(* Logix 5000 AddOnInstructionDefinition export; software revision 16.04 *)

TYPE AKD_Status :   // All connections to the drive ethernet module are established and data is successfully transferring.
STRUCT
   Profile_In_Progress : BOOL;   // Profile Move In Progress
   Block_In_Execution : BOOL;   // Block In Execution
   On_Target_Position : BOOL;   // On Target Position (1=Current Position Equals Last Target Position)
   General_Fault : BOOL;   // General Fault
   Current_Direction : BOOL;   // Current Motor Direction (0=Reverse, 1=Forward)
   Home_Level : BOOL;   // Level of Home Input
   Reg_Level : BOOL;   // Level of Registration Input
   Enable : BOOL;   // State of Enable Output
   Fault_Input_Fault : BOOL;   // Fault Input Active
   Fwd_Limit : BOOL;   // Forward Input Active
   Rev_Limit : BOOL;   // Reverse Input Active
   Positive_Limit : BOOL;   // Positive Software Limit Exceeded
   Negative_Limit : BOOL;   // Negative Software Limit Exceeded
   FE_Fault : BOOL;   // Following Error Fault
   Block_Fault : BOOL;   // Block Execution Fault
   Load_Complete : BOOL;   // Command Message Successfully Loaded
END_STRUCT
END_TYPE

TYPE AKD_Axis :   // Axis Data:
STRUCT
   Control : AKD_Control;   // Control bits to send to the drive
   Status : AKD_Status;   // Status bits received from the drive
   Input : AB:ETHERNET_MODULE_SINT_64Bytes:I:0;   // Data from the drive
   Output : AB:ETHERNET_MODULE_SINT_64Bytes:O:0;   // Data to the drive
   ResponseMsgType : SINT;   // Response type contained in latest IO response from drive. Used to check for errors
   CommandTimeout : INT;   // Time to allow for command response from drive. Dependent on scan rate and communicaiton rate
   PositionFeedback : DINT;   // Actual Position Value
   VelocityFeedback : DINT;   // Actual Velocity Value
END_STRUCT
END_TYPE

TYPE AKD_Control :   // Send Explicit Message
STRUCT
   Load_Data_Start_Profile : BOOL;   // Load Command Data / Start Profile Move
   Start_Block : BOOL;   // Execute Command block or block chain
   Incremental : BOOL;   // Incremental Position (0=Absolute, 1=Incremental)
   Direction : BOOL;   // Direction in Velocity Mode (0=Reverse, 1=Forward)
   Smooth_Stop : BOOL;   // Smooth / Controlled Stop w/ Deceleration
   Hard_Stop : BOOL;   // Hard / Immediate Stop
   Reg_Arm : BOOL;   // Arm the Registration Input
   Enable : BOOL;   // Enable Output
END_STRUCT
END_TYPE

ADD_ON_INSTRUCTION AKD_Set_Position   (* revision 2.1, ExecutePrescan, ExecuteEnableInFalse *)
// Set Drive Position
// Revision note:
// Don't error if Command_Timeout preset is 0
VAR_OUTPUT
   DN : BOOL; {visible}   // Command Successful
   ER : BOOL; {visible}   // Error
END_VAR
VAR_IN_OUT
   Axis : AKD_Axis; {required}
END_VAR
VAR_INPUT
   Incremental : BOOL; {visible}   // Position Definition (0=Absolute, 1=Incremental)
   Position : DINT; {required}   // Position Value
END_VAR
VAR_OUTPUT
   PC : BOOL; {visible}   // Process Complete
   IP : BOOL; {visible}   // In Process
END_VAR
VAR
   Response_Bytes : SINT[8];
   OS_LoadStart : BOOL;
   Position_Internal : DINT;   // Scaled Position Value for Drive
   Command_Timeout : TIMER;   // Timeout Timer
   Command_Message_Type : SINT;   // Command Message Type
   Command_Axis_Number : SINT;   // Command Axis Number
   Response_Message_Type : SINT;   // Response Message Type
   Response_Axis_Number : SINT;   // Response Axis Number
   Command_Bytes : SINT[8];
   Step : SINT;
END_VAR

ROUTINE EnableInFalse   (* ladder *)
// EnableIn_False
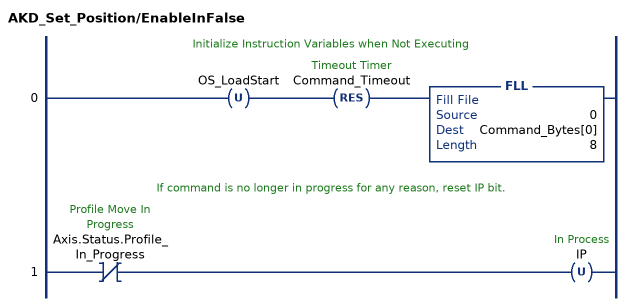
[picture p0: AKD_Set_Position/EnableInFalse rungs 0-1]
   // Initialize Instruction Variables when Not Executing
   0: OTU(OS_LoadStart)RES(Command_Timeout)FLL(0,Command_Bytes[0],8);
   // If command is no longer in progress for any reason, reset IP bit.
   1: XIO(Axis.Status.Profile_In_Progress)OTU(IP);
END_ROUTINE

ROUTINE Logic   (* ladder *)
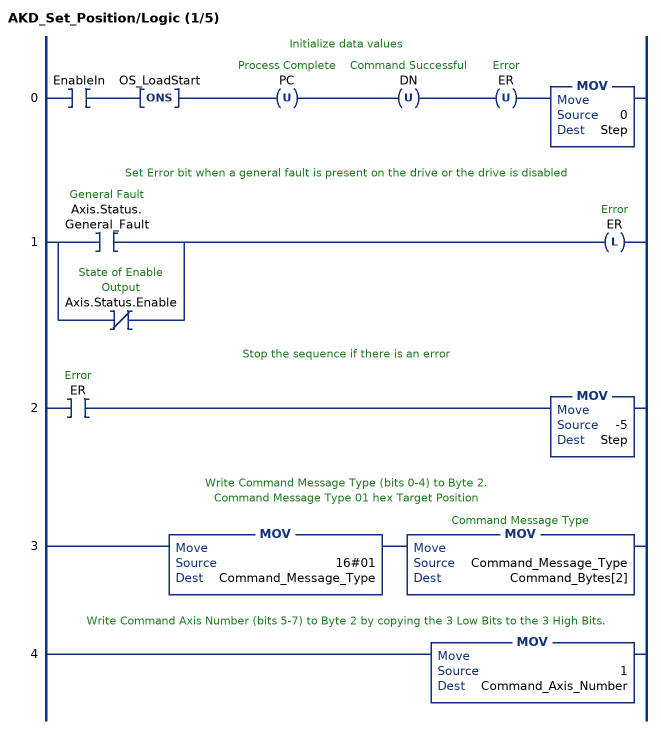
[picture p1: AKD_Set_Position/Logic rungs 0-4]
   // Initialize data values
   0: XIC(EnableIn)ONS(OS_LoadStart)OTU(PC)OTU(DN)OTU(ER)MOV(0,Step);
   // Set Error bit when a general fault is present on the drive or the drive is disabled
   1: [XIC(Axis.Status.General_Fault) ,XIO(Axis.Status.Enable) ]OTL(ER);
   // Stop the sequence if there is an error
   2: XIC(ER)MOV(-5,Step);
   // Write Command Message Type (bits 0-4) to Byte 2.
   // Command Message Type 01 hex Target Position
   3: MOV(16#01,Command_Message_Type)MOV(Command_Message_Type,Command_Bytes[2]);
   // Write Command Axis Number (bits 5-7) to Byte 2 by copying the 3 Low Bits to the 3 High Bits.
   4: MOV(1,Command_Axis_Number);
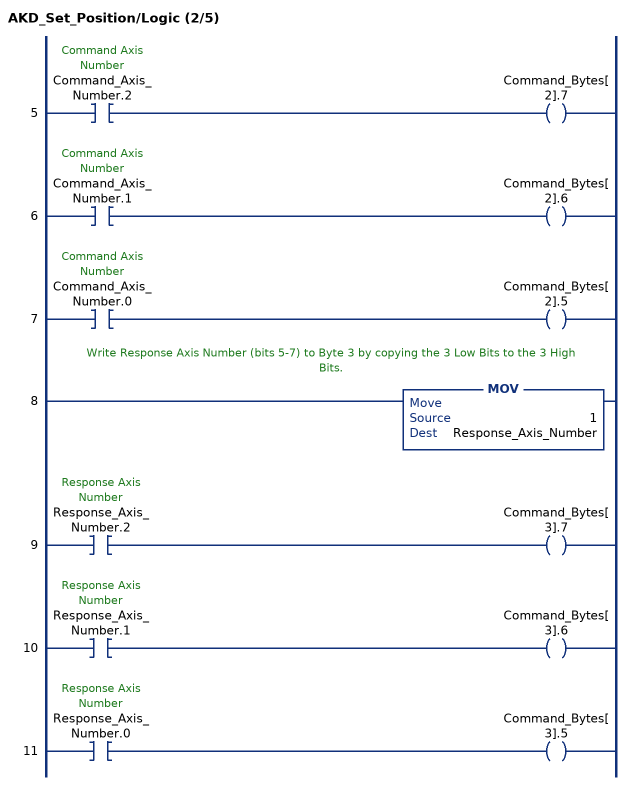
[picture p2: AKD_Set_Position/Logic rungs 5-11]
   5: XIC(Command_Axis_Number.2)OTE(Command_Bytes[2].7);
   6: XIC(Command_Axis_Number.1)OTE(Command_Bytes[2].6);
   7: XIC(Command_Axis_Number.0)OTE(Command_Bytes[2].5);
   // Write Response Axis Number (bits 5-7) to Byte 3 by copying the 3 Low Bits to the 3 High Bits.
   8: MOV(1,Response_Axis_Number);
   9: XIC(Response_Axis_Number.2)OTE(Command_Bytes[3].7);
   10: XIC(Response_Axis_Number.1)OTE(Command_Bytes[3].6);
   11: XIC(Response_Axis_Number.0)OTE(Command_Bytes[3].5);
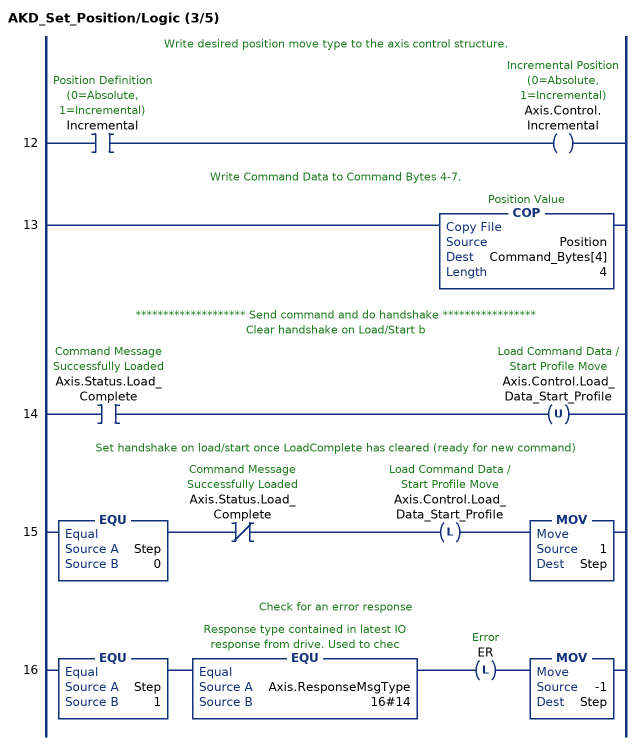
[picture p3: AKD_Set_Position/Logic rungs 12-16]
   // Write desired position move type to the axis control structure.
   12: XIC(Incremental)OTE(Axis.Control.Incremental);
   // Write Command Data to Command Bytes 4-7.
   13: COP(Position,Command_Bytes[4],4);
   // ******************** Send command and do handshake *****************
   // Clear handshake on Load/Start b
   14: XIC(Axis.Status.Load_Complete)OTU(Axis.Control.Load_Data_Start_Profile);
   // Set handshake on load/start once LoadComplete has cleared (ready for new command)
   15: EQU(Step,0)XIO(Axis.Status.Load_Complete)OTL(Axis.Control.Load_Data_Start_Profile)MOV(1,Step);
   // Check for an error response
   16: EQU(Step,1)EQU(Axis.ResponseMsgType,16#14)OTL(ER)MOV(-1,Step);
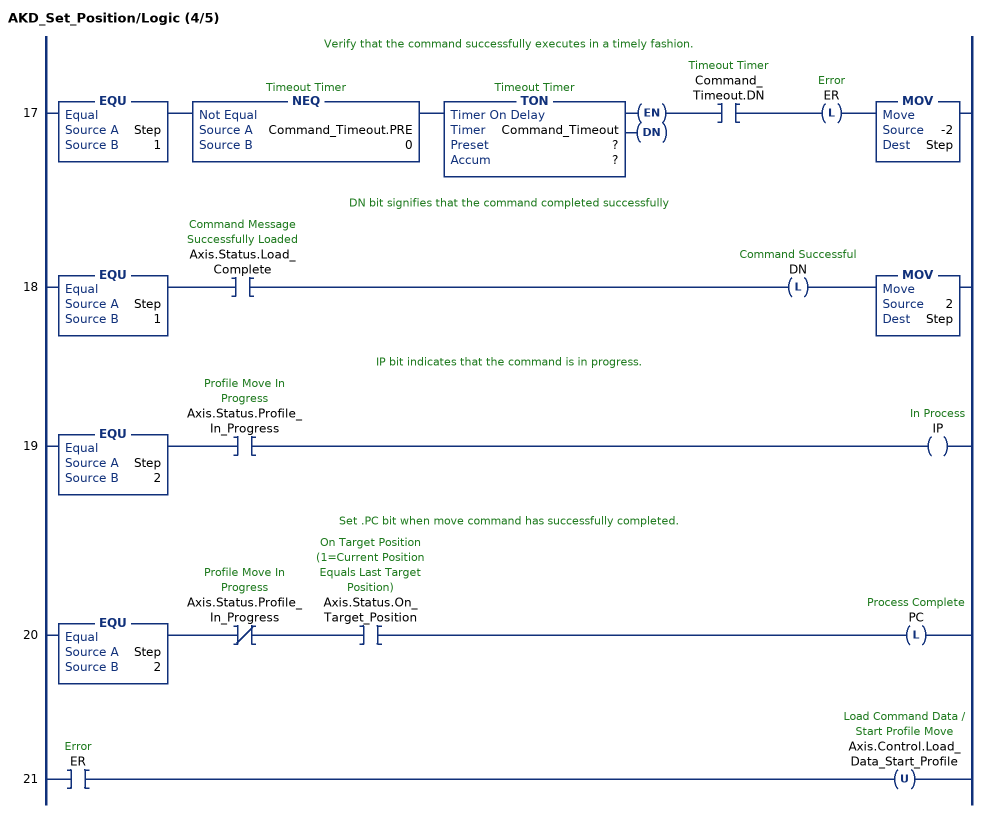
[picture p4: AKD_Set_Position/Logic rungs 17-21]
   // Verify that the command successfully executes in a timely fashion.
   17: EQU(Step,1)NEQ(Command_Timeout.PRE,0)TON(Command_Timeout,?,?)XIC(Command_Timeout.DN)OTL(ER)MOV(-2,Step);
   // DN bit signifies that the command completed successfully
   18: EQU(Step,1)XIC(Axis.Status.Load_Complete)OTL(DN)MOV(2,Step);
   // IP bit indicates that the command is in progress.
   19: EQU(Step,2)XIC(Axis.Status.Profile_In_Progress)OTE(IP);
   // Set .PC bit when move command has successfully completed.
   20: EQU(Step,2)XIO(Axis.Status.Profile_In_Progress)XIC(Axis.Status.On_Target_Position)OTL(PC);
   21: XIC(ER)OTU(Axis.Control.Load_Data_Start_Profile);
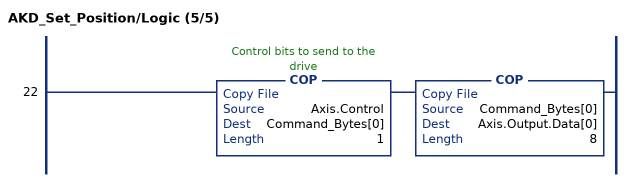
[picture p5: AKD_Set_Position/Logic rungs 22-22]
   22: COP(Axis.Control,Command_Bytes[0],1)COP(Command_Bytes[0],Axis.Output.Data[0],8);
END_ROUTINE

ROUTINE Prescan   (* ladder *)
// Prescan
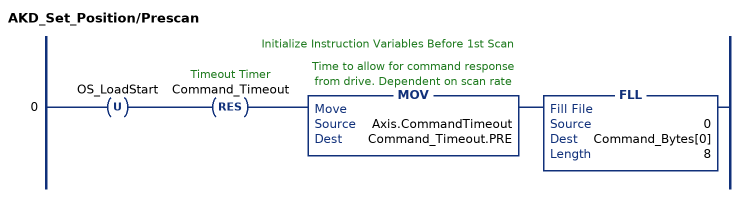
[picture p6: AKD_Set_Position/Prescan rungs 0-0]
   // Initialize Instruction Variables Before 1st Scan
   0: OTU(OS_LoadStart)RES(Command_Timeout)MOV(Axis.CommandTimeout,Command_Timeout.PRE)FLL(0,Command_Bytes[0],8);
END_ROUTINE
END_ADD_ON_INSTRUCTION
